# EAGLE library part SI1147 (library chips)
SENSOR DGTL UV INDEX 10QFN
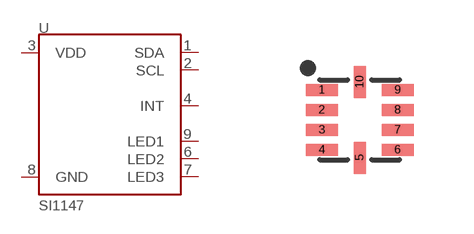
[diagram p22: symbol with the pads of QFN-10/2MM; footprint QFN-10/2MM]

Designator prefix U

## SI1147 (DIGIKEY: 336-2624-1-ND)  [QFN-10/2MM]
1  SDA
2  SCL
3  VDD
4  INT
6  LED2
7  LED3
8  GND
9  LED1

## Footprint QFN-10/2MM (pad centres in mm)
smd 0.8 x 0.3: 1 -0.95,0.75; 2 -0.95,0.25; 3 -0.95,-0.25; 4 -0.95,-0.75; 6 0.95,-0.75; 7 0.95,-0.25; 8 0.95,0.25; 9 0.95,0.75
smd 0.3 x 0.8: 5 0,-0.95; 10 0,0.95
